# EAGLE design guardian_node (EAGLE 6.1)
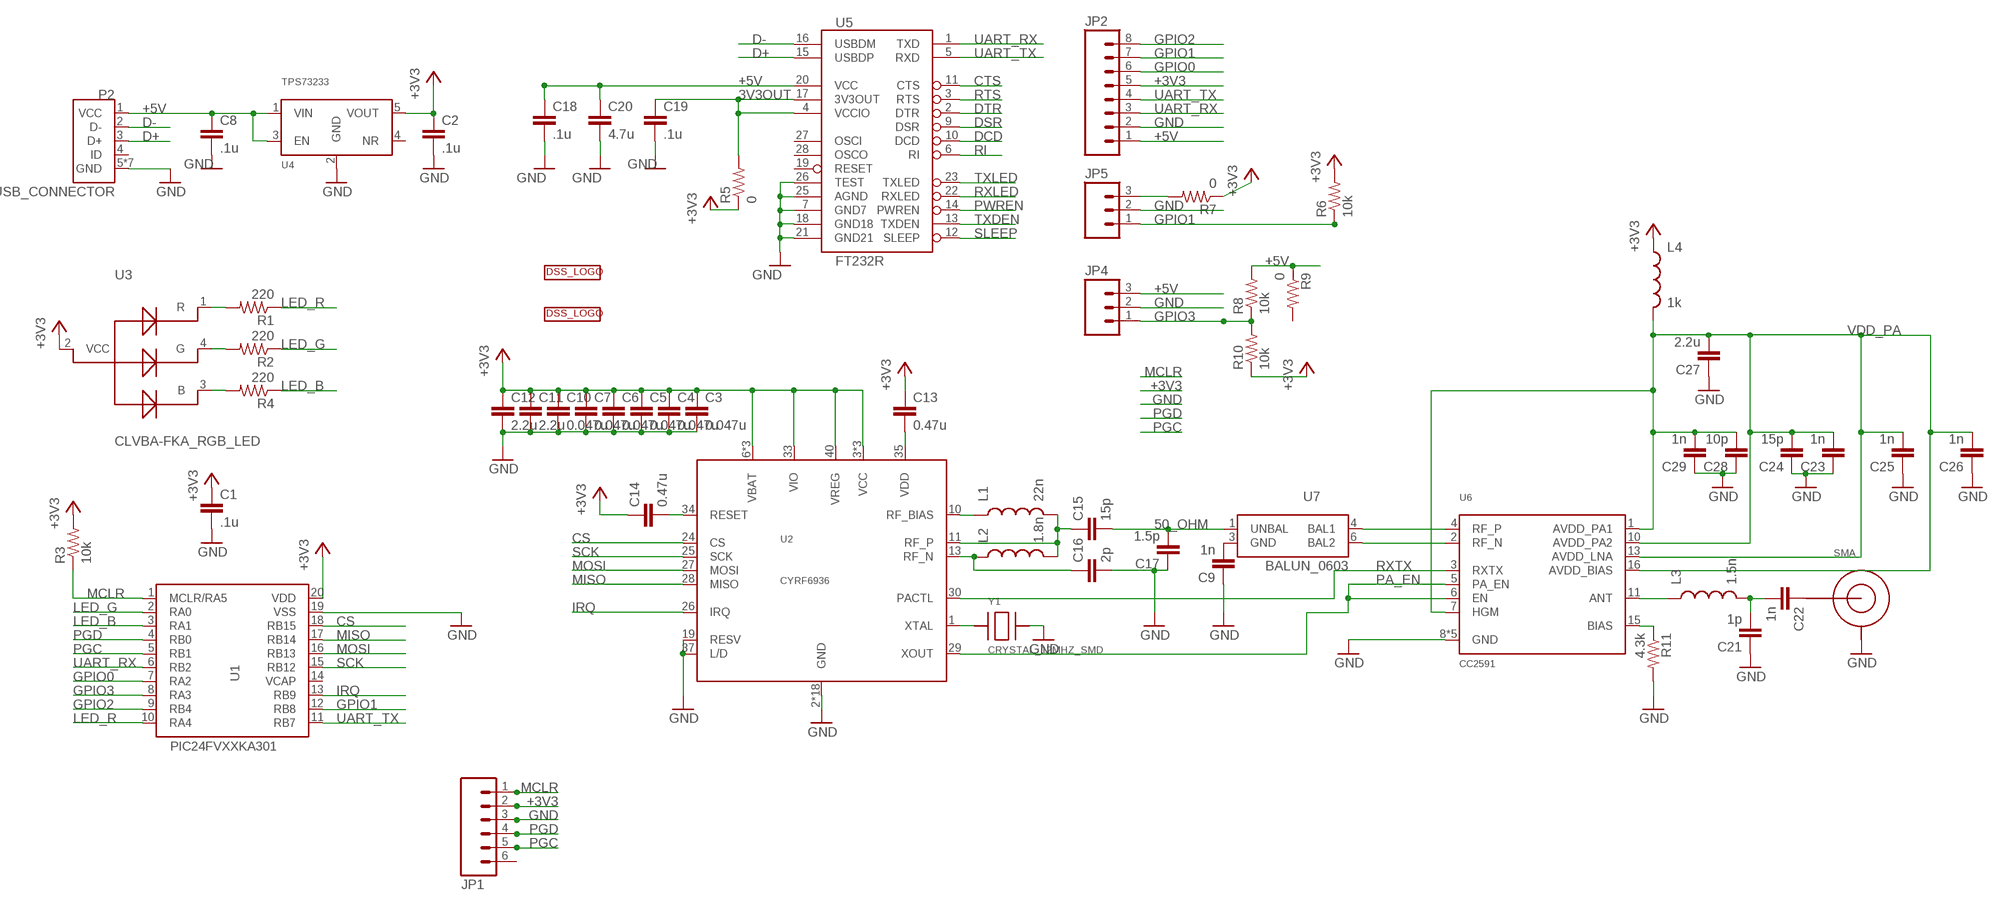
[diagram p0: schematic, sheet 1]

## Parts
C1  .1u  CAP0603-CAP  [0603-CAP]
C2  .1u  CAP0603-CAP  [0603-CAP]
C3  0.047u  CAP0402-CAP  [0402-CAP]
C4  0.047u  CAP0402-CAP  [0402-CAP]
C5  0.047u  CAP0402-CAP  [0402-CAP]
C6  0.047u  CAP0402-CAP  [0402-CAP]
C7  0.047u  CAP0402-CAP  [0402-CAP]
C8  .1u  CAP0603-CAP  [0603-CAP]
C9  1n  CAP0402-CAP  [0402-CAP]
C10  0.047u  CAP0402-CAP  [0402-CAP]
C11  2.2u  CAP0402-CAP  [0402-CAP]
C12  2.2u  CAP0402-CAP  [0402-CAP]
C13  0.47u  CAP0402-CAP  [0402-CAP]
C14  0.47u  CAP0402-CAP  [0402-CAP]
C15  15p  CAP0402-CAP  [0402-CAP]
C16  2p  CAP0402-CAP  [0402-CAP]
C17  1.5p  CAP0402-CAP  [0402-CAP]
C18  .1u  CAP0603-CAP  [0603-CAP]
C19  .1u  CAP0603-CAP  [0603-CAP]
C20  4.7u  CAP0603-CAP  [0603-CAP]
C21  1p  CAP0402-CAP  [0402-CAP]
C22  1n  CAP0402-CAP  [0402-CAP]
C23  1n  CAP0402-CAP  [0402-CAP]
C24  15p  CAP0402-CAP  [0402-CAP]
C25  1n  CAP0402-CAP  [0402-CAP]
C26  1n  CAP0402-CAP  [0402-CAP]
C27  2.2u  CAP0402-CAP  [0402-CAP]
C28  10p  CAP0402-CAP  [0402-CAP]
C29  1n  CAP0402-CAP  [0402-CAP]
JP1  M06SIP  [1X06]
JP2  M081X08  [1X08]
JP4  M03PTH  [1X03]
JP5  M03PTH  [1X03]
L1  22n  INDUCTOR0603  [0603]
L2  1.8n  INDUCTOR0402  [C0402]
L3  1.5n  INDUCTOR0402  [C0402]
L4  1k  INDUCTOR0402  [C0402]
P2  USB_CONNECTOR  [USB_MICRO]
R1  220  RESISTOR0402-RES  [0402-RES]
R2  220  RESISTOR0402-RES  [0402-RES]
R3  10k  RESISTOR0603-RES  [0603-RES]
R4  220  RESISTOR0402-RES  [0402-RES]
R5  0  RESISTOR0603-RES  [0603-RES]
R6  10k  RESISTOR0603-RES  [0603-RES]
R7  0  RESISTOR0603-RES  [0603-RES]
R8  10k  RESISTOR0603-RES  [0603-RES]
R9  0  RESISTOR0603-RES  [0603-RES]
R10  10k  RESISTOR0603-RES  [0603-RES]
R11  4.3k  RESISTOR0402-RES  [0402-RES]
SMA  SMA_PTH  [SMA_PTH]
U1  PIC24FVXXKA301  [SSOP20]
U2  CYRF6936  [QFN40-6X6]
U3  CLVBA-FKA_RGB_LED  [PLCC-4]
U4  TPS73233  [SOT23-5]
U5  FT232R  FT232RLSSOP  [SSOP28DB]
U6  CC2591  [QFN16-4X4]
U7  BALUN_0603  [0603_BALUN]
U$1  DSSBOTTOM  [DSS_BOT]
U$2  DSSTOP  [DSS]
Y1  CRYSTAL_12MHZ_SMD  [SMD-4_5X3.2MM]

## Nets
3V3OUT: C19.1 R5.2 U5.4(VCCIO) U5.17(3V3OUT)
50_OHM: C15.2 C17.2 U7.1(UNBAL)
+3V3: C1.1 C2.1 C3.1 C4.1 C5.1 C6.1 C7.1 C10.1 C11.1 C12.1 C13.1 C14.1 JP1.2 JP2.5 L4.1 R3.2 R5.1 R6.2 R7.1 R10.1 U1.20(VDD) U2.3(VCC) U2.6(VBAT) U2.7(VCC) U2.8(VBAT) U2.16(VCC) U2.33(VIO) U2.38(VBAT) U2.40(VREG) U3.2(VCC) U4.5(VOUT)
+5V: C8.1 C18.1 C20.1 JP2.1 JP4.3 P2.1(VCC) R8.2 R9.1 U4.1(VIN) U4.3(EN) U5.20(VCC)
CS: U1.18(RB15) U2.24(CS)
CTS: U5.11(CTS)
D+: P2.3(D+) U5.15(USBDP)
D-: P2.2(D-) U5.16(USBDM)
DCD: U5.10(DCD)
DSR: U5.9(DSR)
DTR: U5.2(DTR)
GND: C1.2 C2.2 C3.2 C4.2 C5.2 C6.2 C7.2 C8.2 C9.1 C10.2 C11.2 C12.2 C16.2 C17.1 C18.2 C19.2 C20.2 C21.1 C23.1 C24.1 C25.1 C26.1 C27.1 C28.1 C29.1 JP1.3 JP2.2 JP4.2 JP5.2 P2.5(GND) P2.GND1(GND) P2.GND2(GND) P2.GND3(GND) P2.GND4(GND) P2.GND5(GND) P2.GND6(GND) R11.2 SMA.GND1(SHIELD) SMA.GND2(SHIELD) SMA.GND3(SHIELD) SMA.GND4(SHIELD) U1.19(VSS) U2.2(GND) U2.4(GND) U2.5(GND) U2.9(GND) U2.12(GND) U2.14(GND) U2.15(GND) U2.17(GND) U2.18(GND) U2.19(RESV) U2.20(GND) U2.21(GND) U2.22(GND) U2.23(GND) U2.31(GND) U2.32(GND) U2.36(GND) U2.37(L/D) U2.39(GND) U2.EXP(GND) U4.2(GND) U5.7(GND7) U5.18(GND18) U5.21(GND21) U5.25(AGND) U5.26(TEST) U6.8(GND) U6.9(GND) U6.12(GND) U6.14(GND) U6.EXP(GND) Y1.P$3
GPIO0: JP2.6 U1.7(RA2)
GPIO1: JP2.7 JP5.1 R6.1 U1.12(RB8)
GPIO2: JP2.8 U1.9(RB4)
GPIO3: JP4.1 R8.1 R10.2 U1.8(RA3)
IRQ: U1.13(RB9) U2.26(IRQ)
LED_B: R4.1 U1.3(RA1)
LED_G: R2.1 U1.2(RA0)
LED_R: R1.1 U1.10(RA4)
MCLR: JP1.1 R3.1 U1.1(MCLR/RA5)
MISO: U1.17(RB14) U2.28(MISO)
MOSI: U1.16(RB13) U2.27(MOSI)
N$1: R1.2 U3.1(R)
N$2: R2.2 U3.4(G)
N$3: R4.2 U3.3(B)
N$4: JP5.3 R7.2
N$5: L1.1 U2.10(RF_BIAS)
N$6: C15.1 L1.2 L2.2 U2.11(RF_P)
N$7: C13.2 U2.35(VDD)
N$8: C14.2 U2.34(RESET)
N$9: C16.1 L2.1 U2.13(RF_N)
N$10: U2.1(XTAL) Y1.P$1
N$11: U6.4(RF_P) U7.4(BAL1)
N$12: U6.2(RF_N) U7.6(BAL2)
N$13: C22.1 SMA.PIN(CENTER)
N$15: C9.2 U7.3(GND)
N$16: R11.1 U6.15(BIAS)
N$17: L3.1 U6.11(ANT)
N$18: C21.2 C22.2 L3.2
PA_EN: U2.29(XOUT) U6.5(PA_EN) U6.6(EN)
PGC: JP1.5 U1.5(RB1)
PGD: JP1.4 U1.4(RB0)
PWREN: U5.14(PWREN)
RI: U5.6(RI)
RTS: U5.3(RTS)
RXLED: U5.22(RXLED)
RXTX: U2.30(PACTL) U6.3(RXTX)
SCK: U1.15(RB12) U2.25(SCK)
SLEEP: U5.12(SLEEP)
TXDEN: U5.13(TXDEN)
TXLED: U5.23(TXLED)
UART_RX: JP2.3 U1.6(RB2) U5.1(TXD)
UART_TX: JP2.4 U1.11(RB7) U5.5(RXD)
VDD_PA: C23.2 C24.2 C25.2 C26.2 C27.2 C28.2 C29.2 L4.2 U6.1(AVDD_PA1) U6.7(HGM) U6.10(AVDD_PA2) U6.13(AVDD_LNA) U6.16(AVDD_BIAS)
Unconnected: JP1.6 P2.4(ID) R9.2 U1.14(VCAP) U4.4(NR) U5.19(RESET) U5.27(OSCI) U5.28(OSCO)

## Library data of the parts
C1-C29 = SparkFun-Passives:CAP: Capacitor
JP1 = SparkFun-Connectors:M06: Header 6 Standard 6-pin 0.1" header. Use with straight break away headers (SKU : PRT-00116), right angle break away headers (PRT-00553), swiss pins (PRT-00743), machine pins (PRT-00117), and female headers (PRT-00115). Molex polarized connector foot print use with SKU : PRT-08094 with associated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
JP2 = SparkFun-Connectors:M08: Header 8 Standard 8-pin 0.1" header. Use with straight break away headers (SKU : PRT-00116), right angle break away headers (PRT-00553), swiss pins (PRT-00743), machine pins (PRT-00117), and female headers (PRT-00115).
JP4 JP5 = SparkFun-Connectors:M03: Header 3 Standard 3-pin 0.1" header. Use with straight break away headers (SKU : PRT-00116), right angle break away headers (PRT-00553), swiss pins (PRT-00743), machine pins (PRT-00117), and female headers (PRT-00115). Molex polarized connector foot print use with SKU : PRT-08232 with associated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
L1-L4 = SparkFun-Passives:INDUCTOR: Inductors
P2 = DSS:USB_CONNECTOR: USB Connector http://www.digikey.com/product-detail/en/10118192-0001LF/609-4613-1-ND/2785378
R1-R11 = SparkFun-Passives:RESISTOR: Resistor
SMA = DSS:SMA_PTH: SMA through-hole
U1 = DSS:PIC24FVXXKA301: PIC24FVXXKA301
U2 = DSS:CYRF6936: Cypress CYRF6936 2.4GHz DSSS radio. All N/C pins and the exposed pad are tied to ground.
U3 = DSS:CLVBA-FKA_RGB_LED
U4 = DSS:TPS73233: TI TPS73233 - fixed output http://www.ti.com/product/tps73233
U5 = SparkFun:FT232RL: USB UART FT232RL 4th Generation USB UART (USB <-> Serial) Controller. Spark Fun Electronics SKU : COM-00650
U6 = DSS:CC2591: CC2591, 2.4GHz RF Front end
U7 = DSS:BALUN_0603: Balun, 0603 LDB182G4520C-110
U$1 U$2 = DSS:DSS: DSS LOGO
Y1 = DSS:CRYSTAL_12MHZ_SMD: 12MHz crystal, SMD

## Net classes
2 VCC: width 0.406 mm, clearance 0.381 mm

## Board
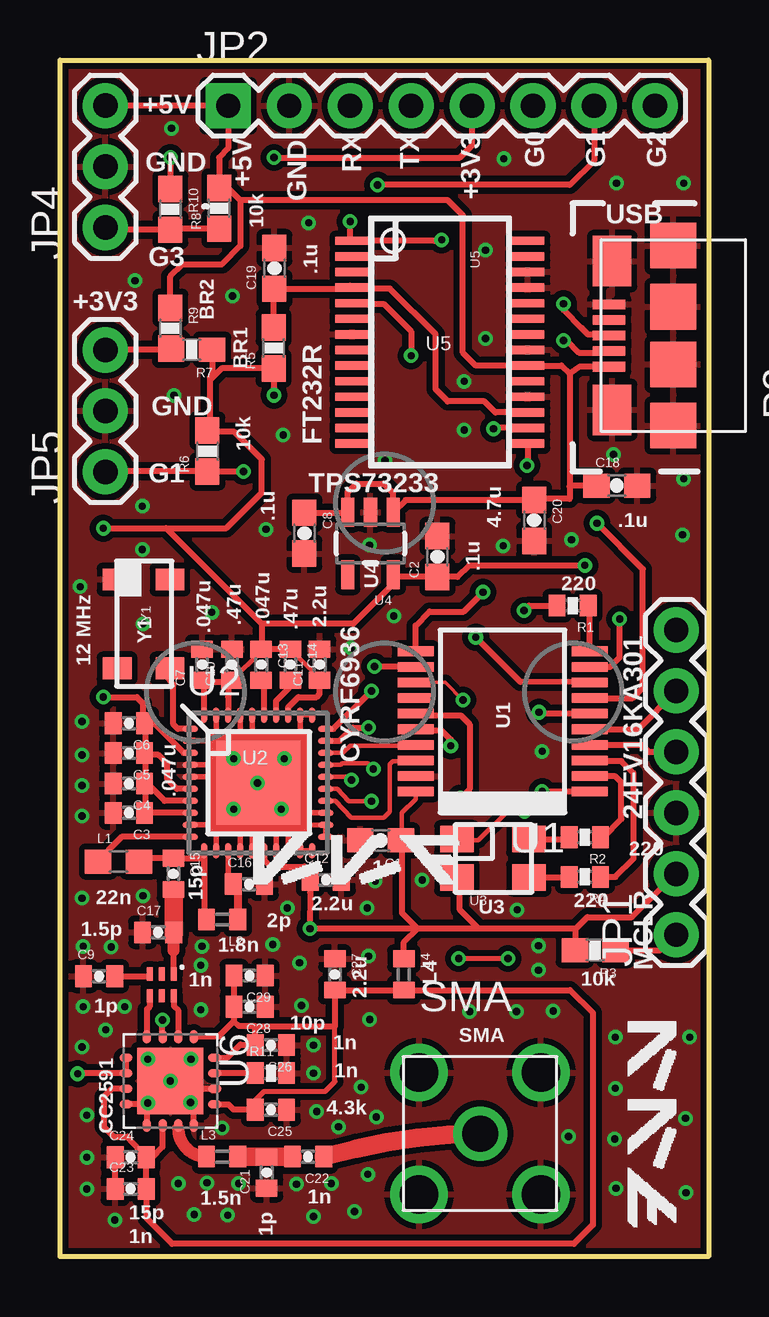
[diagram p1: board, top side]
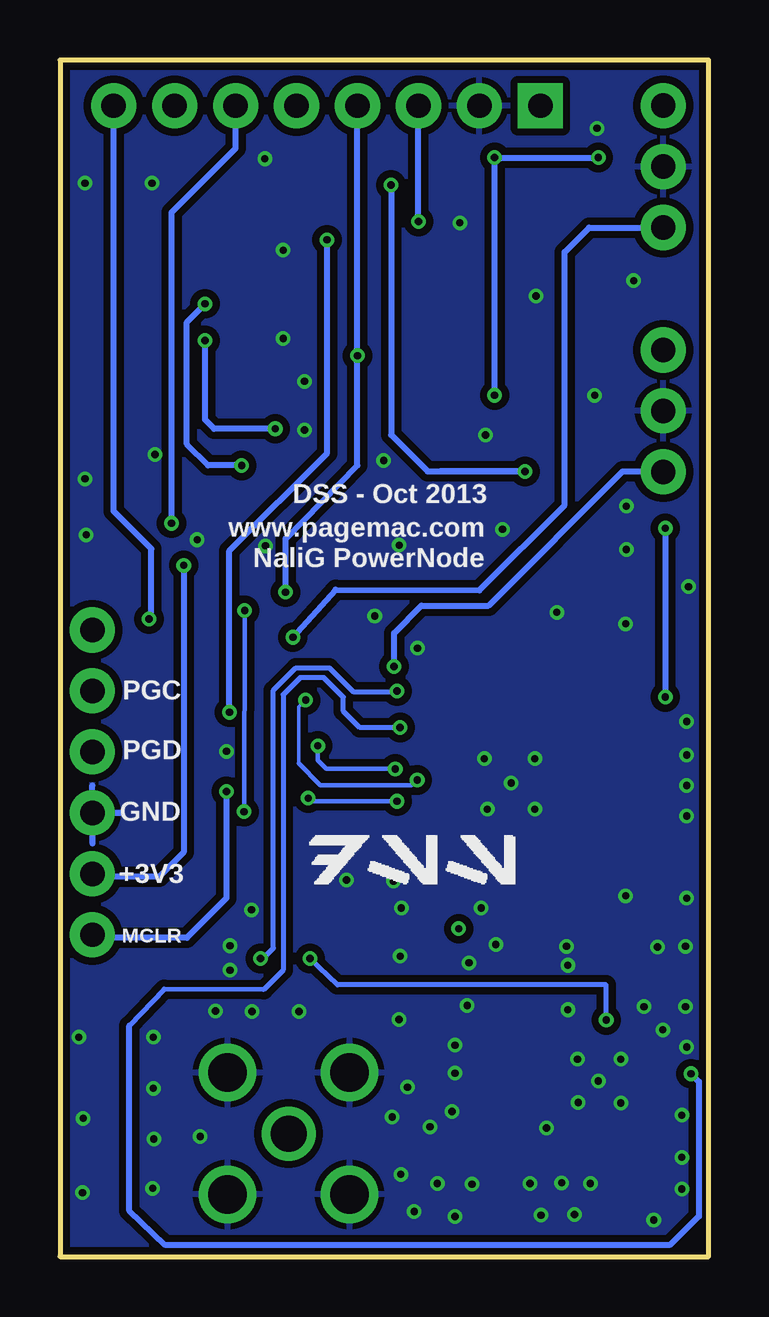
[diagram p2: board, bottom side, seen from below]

Size 27.03 x 49.86 mm. Coordinates in mm from the lower left corner, seen from the top.
Outline: 0,49.86 27.03,49.86 27.03,0 0,0 0,49.86
Copper layers (1*16): Top 0.035mm / dielectric 1.5mm / Bottom 0.035mm
Design rules: minimum track width 6mil, minimum drill 12mil, track to track 6mil, track to pad 6mil, pad to pad 6mil, via to via 6mil, smd to smd 0mil, copper to edge 10mil, drill to drill 10mil, minimum pad ring 10mil, minimum via ring 6mil, stop-mask expansion 2mil, vias tented up to drill 100mil, thermal gap 10mil
tRestrict: area 5.8,3.7 to 11.3,4.6; area 2.3,5.3 to 3.6,6.2; area 6.8,6.5 to 7.8,7.3; area 6.2,14.6 to 7,16.7; area 3.9,17.7 to 5.3,18.5; area 5.5,16.7 to 11.3,22.3; area 5.5,22.9 to 10.4,23.4

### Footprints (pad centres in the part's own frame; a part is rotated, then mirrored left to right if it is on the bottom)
0603-CAP = smd 1.1 x 1: 1 -0.85,0; 2 0.85,0
0402-CAP = smd 0.7 x 0.9: 1 -0.65,0; 2 0.65,0
1X06 = drill 1.016 pad 1.88: 1 0,0; 2 2.54,0; 3 5.08,0; 4 7.62,0; 5 10.16,0; 6 12.7,0
1X08 = drill 1.016 pad 1.88 square: 1 0,0 | drill 1.016 pad 1.88: 2 2.54,0; 3 5.08,0; 4 7.62,0; 5 10.16,0; 6 12.7,0; 7 15.24,0; 8 17.78,0
1X03 = drill 1.016 pad 1.88: 1 0,0; 2 2.54,0; 3 5.08,0
0603 = smd 1.1 x 1: 1 -0.85,0; 2 0.85,0
C0402 = smd 0.7 x 0.9: 1 -0.65,0; 2 0.65,0
USB_MICRO = smd 0.4 x 1.35: 1 -1.3,2.675; 2 -0.65,2.675; 3 0,2.675; 4 0.65,2.675; 5 1.3,2.675 | smd 1.9 x 1.9: GND1 -3.75,0; GND2 -1.2,0; GND3 1.2,0; GND4 3.75,0 | smd 2.1 x 1.6: GND5 -3.1,2.55; GND6 3.1,2.55
0402-RES = smd 0.7 x 0.9: 1 -0.65,0; 2 0.65,0
0603-RES = smd 1.1 x 1: 1 -0.85,0; 2 0.85,0
SMA_PTH = drill 1.6: GND1 2.54,2.54; GND2 -2.54,2.54; GND3 -2.54,-2.54; GND4 2.54,-2.54 | drill 1.5: PIN 0,0
SSOP20 = smd 0.4 x 1.5: 1 -2.925,-3.625; 2 -2.275,-3.625; 3 -1.625,-3.625; 4 -0.975,-3.625; 5 -0.325,-3.625; 6 0.325,-3.625; 7 0.975,-3.625; 8 1.625,-3.625; 9 2.275,-3.625; 10 2.925,-3.625; 11 2.925,3.625; 12 2.275,3.625; 13 1.625,3.625; 14 0.975,3.625; 15 0.325,3.625; 16 -0.325,3.625; 17 -0.975,3.625; 18 -1.625,3.625; 19 -2.275,3.625; 20 -2.925,3.625
QFN40-6X6 = smd 0.65 x 0.25: 1 -2.825,2.25; 2 -2.825,1.75; 3 -2.825,1.25; 4 -2.825,0.75; 5 -2.825,0.25; 6 -2.825,-0.25; 7 -2.825,-0.75; 8 -2.825,-1.25; 9 -2.825,-1.75; 10 -2.825,-2.25; 21 2.825,-2.25; 22 2.825,-1.75; 23 2.825,-1.25; 24 2.825,-0.75; 25 2.825,-0.25; 26 2.825,0.25; 27 2.825,0.75; 28 2.825,1.25; 29 2.825,1.75; 30 2.825,2.25 | smd 0.25 x 0.65: 11 -2.25,-2.825; 12 -1.75,-2.825; 13 -1.25,-2.825; 14 -0.75,-2.825; 15 -0.25,-2.825; 16 0.25,-2.825; 17 0.75,-2.825; 18 1.25,-2.825; 19 1.75,-2.825; 20 2.25,-2.825; 31 2.25,2.825; 32 1.75,2.825; 33 1.25,2.825; 34 0.75,2.825; 35 0.25,2.825; 36 -0.25,2.825; 37 -0.75,2.825; 38 -1.25,2.825; 39 -1.75,2.825; 40 -2.25,2.825 | smd 3.5 x 3.5: EXP 0,0
PLCC-4 = smd 1.4 x 1.1: 1 -1.524,0.812; 2 -1.524,-0.788; 3 1.476,-0.788; 4 1.476,0.812
SOT23-5 = smd 0.55 x 1.2: 1 -0.95,-1.3; 2 0,-1.3; 3 0.95,-1.3; 4 0.95,1.3; 5 -0.95,1.3
SSOP28DB = smd 0.348 x 1.397: 1 -4.225,-3.656; 2 -3.575,-3.656; 3 -2.925,-3.656; 4 -2.275,-3.656; 5 -1.625,-3.656; 6 -0.975,-3.656; 7 -0.325,-3.656; 8 0.325,-3.656; 9 0.975,-3.656; 10 1.625,-3.656; 11 2.275,-3.656; 12 2.925,-3.656; 13 3.575,-3.656; 14 4.225,-3.656; 15 4.225,3.656; 16 3.575,3.656; 17 2.925,3.656; 18 2.275,3.656; 19 1.625,3.656; 20 0.975,3.656; 21 0.325,3.656; 22 -0.325,3.656; 23 -0.975,3.656; 24 -1.625,3.656; 25 -2.275,3.656; 26 -2.925,3.656; 27 -3.575,3.656; 28 -4.225,3.656
QFN16-4X4 = smd 0.55 x 0.35: 1 -1.85,0.975; 2 -1.85,0.325; 3 -1.85,-0.325; 4 -1.85,-0.975; 9 1.85,-0.975; 10 1.85,-0.325; 11 1.85,0.325; 12 1.85,0.975 | smd 0.35 x 0.55: 5 -0.975,-1.85; 6 -0.325,-1.85; 7 0.325,-1.85; 8 0.975,-1.85; 13 0.975,1.85; 14 0.325,1.85; 15 -0.325,1.85; 16 -0.975,1.85 | smd 2.76 x 2.76: EXP 0,0
0603_BALUN = smd 0.55 x 0.25: 1 -0.27,1; 2 -0.27,0.5; 3 -0.27,0; 4 0.63,0; 5 0.63,0.5; 6 0.63,1
SMD-4_5X3.2MM = smd 0.9 x 1.2: P$1 1.9,1.1; P$2 1.9,-1.1; P$3 -1.8,-1.1; P$4 -1.8,1.1

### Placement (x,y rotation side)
C1  13.36,17.35 180 top
C2  15.73,29.17 90 top
C3  2.87,18.49 180 top
C4  2.87,19.71 180 top
C5  2.87,20.98 180 top
C6  2.87,22.22 180 top
C7  5.92,24.66 90 top
C8  10.18,30.15 270 top
C9  1.63,11.68 0 top
C10  7.16,24.66 90 top
C11  10.82,24.66 90 top
C12  11.07,15.7 0 top
C13  8.38,24.66 270 top
C14  9.6,24.66 270 top
C15  4.72,15.95 270 top
C16  7.87,15.52 0 top
C17  4.09,13.51 0 top
C18  23.2,32.12 0 top
C19  8.94,41.18 90 top
C20  19.76,30.68 270 top
C21  8.61,3.51 90 top
C22  10.34,4.17 180 top
C23  2.95,2.82 0 top
C24  2.95,4.14 0 top
C25  8.79,6.12 180 top
C26  8.79,8.81 180 top
C27  11.46,11.76 270 top
C28  7.9,10.41 180 top
C29  7.9,11.71 180 top
JP1  25.68,13.41 90 top
JP2  7.01,47.96 0 top
JP4  1.89,42.88 90 top
JP5  1.89,32.7 90 top
L1  2.44,16.46 0 top
L2  6.76,14.05 180 top
L3  6.76,4.17 0 top
L4  14.33,11.76 270 top
P2  25.55,38.38 90 top
R1  21.36,27.13 180 top
R2  21.87,17.48 180 top
R3  22.3,12.78 180 top
R4  21.87,15.82 180 top
R5  8.9,37.86 90 top
R6  6.15,33.57 90 top
R7  5.49,37.8 180 top
R8  6.64,43.68 90 top
R9  4.6,38.68 270 top
R10  4.6,43.64 270 top
R11  8.79,7.65 0 top
SMA  17.5,5.13 0 top
U1  18.44,22.3 90 top
U2  8.25,19.74 0 top
U3  18.06,16.59 0 top
U4  12.94,29.71 180 top
U5  15.83,38.1 270 top
U6  4.6,7.32 270 top
U7  3.73,11.51 270 top
U$1  7.9,15.32 0 top
U$2  25.88,1.07 90 top
Y1  3.48,26.42 270 top

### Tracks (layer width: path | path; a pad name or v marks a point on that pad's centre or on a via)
3V3OUT
  Top 0.254: U5.17 18.14,35.18 17.68,35.64 16.15,35.64 15.65,36.14 15.65,38.43 13.74,40.34 12.22,40.34 | 12.22,40.34 12.09,40.46 | R5.2 8.9,40.3 C19.1 12.12,40.33 U5.4 12.21,40.34 12.22,40.34
50_OHM
  Top 0.254: U7.1 4.73,13.46 4.66,13.46 C17.2 | C15.2
  Top 0.762: 4.73,13.46 C15.2
+3V3  (via drill 0.3)
  Top 0.178: U2.33 9.52,22.56 9.55,22.53 | 10.82,24.09 C14.1 | 8.38,25.23 C10.1 | U1.20 14.82,19.06 14.25,18.49 14.25,17.39 C1.1 | 10.44,15.95 C12.1
  Top 0.254: v21.87,28.8 17.04,28.8 16.56,28.32 C2.1 13.98,28.32 U4.5 13.89,28.04 12.22,26.37 8.44,26.37 8.43,26.35 | 3.58,18.49 U2.8 3.59,18.49 3.58,18.49 | U2.7 4.36,18.99 3.71,19.63 3.6,19.63 C4.1 3.57,19.76 3.58,19.76 | 3.45,21.04 C5.1 | U2.38 7.01,23.32 7.04,24.1 C10.1 7.1,23.95 5.99,23.95 6.01,23.94 U2.40 6.01,23.81 5.87,23.95 5.92,24 C7.1 | U2.16 8.51,16.54 8.79,16.26 10.19,16.26 10.44,15.95 | 10.82,24.09 C11.1 10.82,23.44 10.69,23.32 9.93,23.32 9.51,22.89 U2.33 | C14.1 C13.1 | C13.1 8.38,25.23 | 8.41,25.29 8.41,26.37 8.42,26.35 8.43,26.35 | v1.8,23.32 3.2,23.32 3.45,23.06 3.45,22.29 C6.1 3.57,22.17 3.58,22.17 | U2.6 4.87,19.49 4.47,19.89 4.47,20.52 4.09,20.9 3.45,20.9 3.45,20.92 C5.1 | U2.3 5.15,20.99 3.96,22.17 3.58,22.17 | 3.45,18.36 3.58,18.49 | C3.1 3.58,18.49 | 3.58,18.49 3.58,19.76 | 3.58,19.76 3.58,21.03 | 3.58,21.03 3.58,22.17 | C5.1 3.53,20.98 3.58,21.03 | 8.41,25.22 8.41,25.29 | 8.41,25.29 C13.1 | 16.43,15.7 U3.2 | JP1.2 23.83,14.15 21.97,14.15 21.49,13.67 | U3.2 16.66,15.67 16.66,14.45 17.45,13.67 | 16.51,15.82 U3.2 | 14.25,17.39 14.25,14.33 14.91,13.67 | 21.49,13.67 17.45,13.67 | 17.45,13.67 14.91,13.67 | 14.91,13.67 v10.41,13.67 10.42,15.17 C12.1 | v1.8,30.35 4.42,30.35 | 4.42,30.35 8.43,26.35 | 6.25,36.53 6.25,36.65 6.34,36.74 R7.1 | 6.25,36.53 6.25,34.49 6.17,34.42 R6.2 6.2,34.42 6.25,34.37 7.26,34.37 8.41,33.22 8.41,31.83 6.93,30.35 4.42,30.35 | 6.25,36.53 6.73,37.01 R5.1 8.9,35.9 v8.92,35.89 | v8.92,45.8 16.66,45.8 17.17,46.3 JP2.5 | v4.6,45.8 R10.1 | 21.49,13.67 21.49,12.81 R3.2 | L4.1 14.33,13.11 14.91,13.67
  Bottom 0.254: v21.87,28.8 21.87,16.84 22.89,15.82 25.55,15.82 JP1.2 | v1.8,30.35 v1.8,23.32 | v8.92,35.89 v8.92,45.8 v4.6,45.8
+5V
  Top 0.254: C8.1 11.97,31 U4.3 11.99,31.85 12.34,32.21 13.49,32.21 13.87,31.83 13.87,31.06 | 13.87,31.06 13.87,31.03 U4.1 14.4,31.53 C20.1 19.81,31.57 21.23,31.57 21.23,32.08 | P2.1 21.66,37.08 21.23,36.78 | 21.23,36.78 21.23,32.08 | 14,30.94 13.87,31.06 | 21.23,36.78 20.89,37.13 U5.20 17.33,37.13 16.79,37.67 16.79,43.38 16.15,44.02 7.52,44.02 | JP4.3 JP2.1 7.01,46.18 6.63,45.8 R8.2 7.01,44.53 7.52,44.02 | C18.1 21.28,32.12 21.23,32.08 | R9.1 4.6,40.84 5.11,41.35 6.76,41.35 7.52,42.11 7.52,44.02
CS
  Top 0.178: U2.24 11.47,18.99 12.14,18.29 13.49,18.29 13.74,18.54 13.74,20.52 13.87,20.65 14.79,20.65
  Top 0.254: 14.79,20.65 U1.18
D+  (via drill 0.3)
  Top 0.254: U5.15 19.48,32.99 v19.46,32.97 | v20.98,39.7 20.98,39.45 21.74,38.68 22,38.43 22.83,38.43 P2.3
  Bottom 0.254: v19.46,32.97 20.85,32.97 21.74,33.86 21.74,38.94 v20.98,39.7
D-  (via drill 0.3)
  Top 0.254: U5.16 18.09,34.53 v18.06,34.49 | v20.98,38.18 21.11,38.18 21.62,37.67 22.82,37.67 P2.2
  Bottom 0.254: v18.06,34.49 20.6,34.49 20.98,34.87 v20.98,38.18
GND  (via drill 0.3)
  Top 0.178: 6.51,17.91 6.86,18.26 v7.24,18.64 | 9.01,17.96 9.01,18.16 | 9.01,18.16 9.01,18.56 v9.22,18.64 | 8.01,18.06 8.08,18.14 8.08,18.06 8.9,18.06 9.01,18.16 | 6.97,20.49 7.47,20.47 | 7.47,20.47 7.04,20.9 7.04,21.23 6.78,21.49 6.55,21.49 6.51,21.53 | 7.51,21.53 7.65,21.39 7.65,21.13 7.32,20.8 7.26,20.75 | 8.01,21.52 7.26,20.78 7.47,20.47 | 10.01,21.54 v9.35,20.75 | 10.03,22.56 U2.31 | U2.31 | U2.31
  Top 0.229: U2.9 6.58,17.99 | U2.12 6.51,17.91 | U2.17 9.01,17.96 | U2.15 8.01,18.06 | U2.14 7.51,18.38 | U2.2 6.55,21.49 | U2.39 6.51,21.53 | U2.37 7.51,21.53 | U2.36 8.01,21.52 | 10.01,21.54 U2.32 10.03,22.56 | U2.4 6.97,20.49 | U2.5 7.98,19.99 | U2.18 9.51,17.93 | U2.20 U2.19 10.01,18.49 11.13,18.49 | 9.81,17.98 U2.22 U2.21 | 7.26,20.78 7.26,20.8 7.32,20.8 7.32,20.83 7.19,20.83 | 7.26,20.75 7.26,20.85 7.29,20.85 7.29,20.83 6.93,20.83 6.93,19.66 8.23,19.66
  Top 0.254: 6.97,20.49 7.26,20.78 | 6.58,17.99 6.86,18.26 | C23.1 C24.1 | U6.14 4.98,6.99 | 4.98,6.99 4.92,6.99 U6.EXP | 4.98,6.99 5.44,6.53 v5.44,6.43 5.57,6.43 U6.12 | U6.8 3.62,6.34 v3.66,6.4 3.67,6.4 U6.9 | v8.23,19.74 8.2,19.74 7.47,20.47 | 7.98,19.99 arc-90 v8.23,19.74 | v7.24,18.64 arc90 7.51,18.38 | 10.01,18.49 10.01,18.64 v9.22,18.64 arc-90 9.51,18.36 9.51,17.93 9.81,17.98 | U2.23 11.13,18.49 | v8.23,19.74 U2.EXP | U2.22 11.05,17.98
  Bottom 0.254: JP1.3 24.46,18.49 | JP1.3 25.68,19.63 | JP1.3 25.68,17.22
  other vias: 3.43,29.46 6.32,26.85 15.09,15.7 0.91,22.3 8.86,13 0.97,12.93 0.91,14.94 5.92,12.93 25.93,30.07 0.91,20.9 0.91,19.63 0.91,18.36 3.45,15.04 19.94,11.94 19.94,12.95 0.84,27.91 3.45,26.37 21.31,29.87 19.05,14.45 3.43,31.27 4.75,35.89 12.9,29.64 9.3,34.24 8.59,30.3 18.47,29.62 16.84,34.44 23.19,44.73 13.54,33.17 25.98,44.73 25.98,32.41 20.09,21.06 12.85,12.52 17.73,41.94 3.12,40.67 7.19,40.03 4.65,47.02 23.06,33.43 18.49,45.75 10.36,43.08 16.84,36.47 17.73,38.25 13.13,15.65 3.66,8.23 5.46,8.23 9.47,14.53 2.13,12.9 5.87,10.29 2.69,10.41 0.97,10.41 5.87,12.14 4.93,3.05 6.12,3.07 7.44,3.05 9.86,3.02 6.76,5.36 11.61,5.41 13.18,5.82 11.3,3.05 10.57,7.65 10.57,8.81 10.57,1.68 1.12,4.14 1.12,2.82 6.99,1.73 12.83,3.43 10.69,6.05 12.9,9.88 17.07,10.21 26.09,2.67 26.24,9.14 19.02,10.21 12.8,14.53 9.98,12.24 10.06,10.46 1.12,5.89 0.91,8.74 1.91,9.45 26.06,5.77 5.59,1.75 23.14,7.01 23.16,2.84 23.11,4.9 21.18,5 20.55,10.24 23.14,9.14 2.29,1.52 13.91,26.7 12.13,25.35 12.27,1.88 7.24,20.75 4.6,7.32 12.55,7.06
  pour Top (isolate 0.254): -0.36,50.36 27.22,50.5 26.97,-0.13 0.03,-0.15
  pour Bottom (isolate 0.305): -0.05,-0.23 26.87,-0.23 27.2,50.5 -0.33,50.31
GPIO0  (via drill 0.3)
  Top 0.254: U1.7 23.86,23.28 24.28,23.7 24.28,28.65 v22.38,30.56
  Bottom 0.254: v22.38,30.56 22.38,43.51 19.71,46.18 JP2.6
GPIO1  (via drill 0.3)
  Top 0.254: U1.12 13.12,24.58 v13.11,24.59 | JP5.1 1.91,32.72 R6.1 v7.65,32.72 | JP2.7 22.25,45.67 21.23,44.65 v13.23,44.65 | v7.65,32.72
  Bottom 0.254: v13.11,24.59 13.11,25.98 11.96,27.13 9.17,27.13 3.58,32.72 1.93,32.72 1.91,32.72 JP5.1 | v13.23,44.65 13.23,34.24 11.71,32.72 11.2,32.72 | 11.2,32.72 v7.65,32.72 11.2,32.72
GPIO2  (via drill 0.3)
  Top 0.254: U1.9 22.93,24.58 23.32,24.97 v23.32,26.57
  Bottom 0.254: v23.32,26.57 23.22,26.62 23.22,29.49 24.79,31.06 JP2.8
GPIO3  (via drill 0.3)
  Top 0.254: U1.8 19.18,23.95 v17.32,25.81 | R8.1 4.64,42.83 R10.2 2.02,42.79 1.93,42.88 JP4.1
  Bottom 0.254: v17.32,25.81 15.54,27.79 9.55,27.76 5.99,31.32 5.99,41.86 4.98,42.88 JP4.1
IRQ  (via drill 0.3)
  Top 0.152: U1.13 16.05,23.93 v16.79,23.19
  Top 0.178: U2.26 12.02,19.99 v12.14,19.86
  Bottom 0.152: 17.07,20.55 17.07,22.91 v16.79,23.19
  Bottom 0.178: 17.07,20.55 16.18,19.63 12.4,19.63 v12.14,19.86
LED_B
  Top 0.254: R4.1 23.14,15.82 23.9,16.59 23.9,20.14 23.39,20.65 22.09,20.65 U1.3
LED_G
  Top 0.254: R2.1 22.63,17.48 23.39,18.24 23.39,19.76 23.14,20.02 22.08,20.02 U1.2
LED_R
  Top 0.254: U1.10 22.07,27.07 R1.1
MCLR  (via drill 0.3)
  Top 0.254: U1.1 v20.1,19.38 v20.09,19.38 | R3.1 25.02,12.78 JP1.1
  Bottom 0.254: v20.09,19.38 20.09,14.94 21.74,13.28 25.55,13.28 JP1.1
MISO
  Top 0.178: U2.28 11.79,20.99 12.09,21.29 14.77,21.29
  Top 0.254: 14.77,21.29 U1.17
MOSI  (via drill 0.3)
  Top 0.178: U2.27 11.7,20.49 11.76,20.55 12.83,20.55 v13.06,20.32
  Top 0.254: U1.16 14.87,21.92 14.88,21.92 15.9,21.92 16.28,21.54 v16.28,21.29
  Bottom 0.178: v13.06,20.32 15.93,20.32 16.28,20.68 v16.28,21.29
N$1  (via drill 0.3)
  Top 0.178: v19.35,18.54 18.64,18.54 17.42,17.35 16.59,17.35 U3.1
  Top 0.254: v19.33,26.92 19.53,27.13 R1.2
  Bottom 0.178: v19.33,26.92 v19.35,18.54
N$2
  Top 0.254: U3.4 21.4,17.4 R2.2
N$3
  Top 0.254: U3.3 21.45,15.8 R4.2
N$4
  Top 0.254: R7.2 2.03,37.8 | 2.03,37.8 1.91,37.8 JP5.3 | 4.76,37.8 2.03,37.8
N$5
  Top 0.254: U2.10 2.58,17.49 1.42,16.33 1.42,16.37 L1.1
N$6
  Top 0.254: U2.11 6.01,15.7 | 6.01,15.7 6.01,14.18 6.12,14.05 L2.2 | 6.01,15.7 5.99,16.6 C15.1 3.18,16.6 L1.2
N$7
  Top 0.254: U2.35 8.51,23.89 C13.2
N$8
  Top 0.254: U2.34 9.01,23.15 9.55,23.7 9.55,23.96 C14.2
N$9
  Top 0.229: U2.13 7.01,15.74 arc90 C16.1 arc-90 7.41,15.34
  Top 0.254: L2.1 7.29,14.17
  Top 0.33: 7.41,15.34 L2.1
N$10
  Top 0.254: U2.1 4.91,21.99 4.72,22.17 4.72,23.83 4.34,24.33 4.6,24.46 4.58,24.57 Y1.P$1
N$11
  Top 0.254: U7.4 3.73,10.41 3.63,10.31 3.63,10.29 3.62,10.29 U6.4
N$12
  Top 0.254: U7.6 arc90 4.75,10.87 4.75,10.44 4.92,10.27 U6.2
N$13
  Top 0.762: C22.1 12.34,4.5 arc-13 SMA.PIN
N$15
  Top 0.254: C9.2 3.64,11.68 U7.3
N$16
  Top 0.254: R11.1 U6.15
N$17
  Top 0.254: U6.11 4.92,5.35
  Top 0.508: 4.92,5.35 arc90 L3.1
N$18
  Top 0.254: 7.42,4.16 arc-90 L3.2 | C21.2 arc-90 C21.2 C22.2
  Top 0.762: 7.42,4.16 9.68,4.16 C22.2
N$19
  Top 0.508: 4.72,13.36 4.72,12.75
PA_EN  (via drill 0.3)
  Top 0.254: U6.5 U6.6 0.76,7.64 v0.74,7.62 | U2.29 11.66,21.49 12.22,22.05 v12.85,22.05
  Bottom 0.203: v12.85,22.05 14.53,22.05 15.21,22.73 15.21,23.32 16.03,24.13 17.02,24.13 17.73,23.42 17.73,11.94 18.54,11.13 22.68,11.15 24.13,9.63
  Bottom 0.254: 24.13,9.63 24.13,1.91 22.63,0.48 1.63,0.48 0.41,1.68 0.41,7.29 v0.74,7.62
PGC
  Top 0.254: U1.5 24.08,21.98 JP1.5
PGD
  Top 0.254: U1.4 24.24,21.33 24.54,21.03 JP1.4
RXTX  (via drill 0.3)
  Top 0.203: v18.67,12.42 v16.61,12.42
  Top 0.254: U6.3 arc-90 4.27,9.22 v4.27,9.86 | U2.30 11.39,21.99 v12.98,23.57
  Bottom 0.203: v4.27,9.86 4.27,11.33 15.47,11.33 v16.61,12.42 | v12.98,23.57 13,23.55 14.81,23.55 15.8,24.54 17.2,24.54 18.14,23.6 18.14,12.85 18.57,12.42 v18.67,12.42
SCK  (via drill 0.3)
  Top 0.178: U2.25 11.55,19.49 12.04,18.97 v12.98,18.97
  Top 0.254: U1.15 14.89,22.56 16.69,22.56 17.07,22.17 17.07,19.48 v16.69,19.1
  Bottom 0.178: v12.98,18.97 16.51,18.97 16.66,19.13 v16.69,19.1
UART_RX  (via drill 0.3)
  Top 0.254: U1.6 19.96,22.63 v19.96,22.68 | v15.9,42.37 15.61,42.33 U5.1 12.09,42.41 v12.09,43.13
  Bottom 0.254: v19.96,22.68 19.96,29.41 15.9,33.48 v15.9,42.37 | 12.09,48.08 JP2.3 v12.09,43.13
UART_TX  (via drill 0.3)
  Top 0.254: U1.11 14.82,26.3 15.39,26.87 16.81,26.87 v17.63,27.69 | U5.5 12.2,39.7 13.49,39.7 14.63,38.56 v14.63,37.54
  Bottom 0.254: v17.63,27.69 17.63,29.92 14.63,32.97 v14.63,37.54 JP2.4
VDD_PA
  Top 0.203: C25.2 8.14,6.51 8.51,6.88 11.05,6.88 11.46,7.29 11.46,9.6
  Top 0.254: U6.10 4.27,4.57 3.84,4.14 C24.2 | 7.25,9.82 C28.2 C29.2 | 7.25,9.82 6.6,9.17 U6.1 | 8.13,9.6 7.46,9.6 7.25,9.82 | U6.16 6.97,8.29 7.52,8.84 8.11,8.84 | 8.11,8.84 C26.2 | 8.11,8.84 8.13,8.84 8.13,9.6 | U6.13 7.02,6.34 7.24,6.12 C25.2 | C24.2 C23.2 3.61,2.81 3.61,1.6 4.67,0.53 21.41,0.53 22.2,1.32 22.2,10.16 21.25,11.11 L4.2 C27.2 | U6.7 2.16,6.99 1.83,6.66 1.83,5.41 2.24,5 2.81,5 C24.2 | 8.13,9.6 11.46,9.6 C27.2 | C27.2 11.46,11.13 11.58,11.13 C27.2
(copper drawn outside any net)
  shapes: Top area x1

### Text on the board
tDocu: B0 | B3 | B4 | B2 | B1
_tsilk: +5V | +5V | GND | RX | TX | +3V3 | G0 | G1 | G2 | GND | 10k | USB | G3 | .1u | +3V3 | BR2 | FT232R | U5 | BR1 | GND | 10k | G1 | TPS73233 | 4.7u | .1u | .1u | .1u | .047u | 220 | 12 MHz | .47u | U4 | Y1 | 2.2u | .047u | .47u | 24FV16KA301 | U1 | .047u | U2 | CYRF6936 | 220 | 15p | .1u | 220 | 22n | 2.2u | U3 | 1.5p | 1.8n | 2p | 1n | L4 | 10k | MCLR | 1p | 2.2u | 10p | 1n | SMA | 1n | 4.3k | CC2591 | 1.5n | 1n | 15p | 1n | 1p
_bsilk: DSS - Oct 2013 | www.pagemac.com | NaliG PowerNode | PGC | PGD | GND | +3V3 | MCLR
